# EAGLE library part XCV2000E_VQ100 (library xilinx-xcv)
xcv2000e_vq100 edit this description Auto generated by make-symbol-device-package-bsdl.ulp Rev. 26 Source: xcv2000e_vq100.bsd
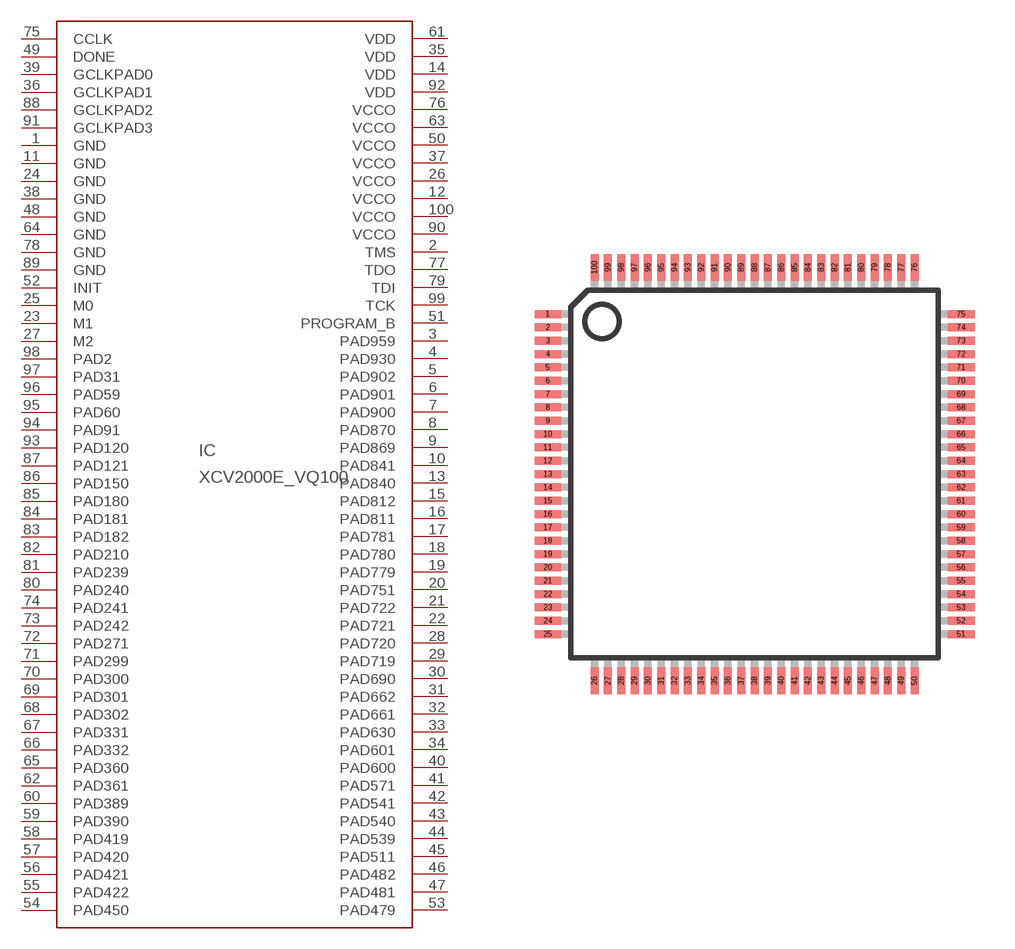
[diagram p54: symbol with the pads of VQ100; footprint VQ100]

Designator prefix IC

## XCV2000E_VQ100 (OC_FARNELL: unknown; OC_NEWARK: unknown)  [VQ100]
1  GND  pwr
2  TMS  in
3  PAD959
4  PAD930
5  PAD902
6  PAD901
7  PAD900
8  PAD870
9  PAD869
10  PAD841
11  GND  pwr
12  VCCO  pwr
13  PAD840
14  VDD  pwr
15  PAD812
16  PAD811
17  PAD781
18  PAD780
19  PAD779
20  PAD751
21  PAD722
22  PAD721
23  M1  in
24  GND  pwr
25  M0  in
26  VCCO  pwr
27  M2  in
28  PAD720
29  PAD719
30  PAD690
31  PAD662
32  PAD661
33  PAD630
34  PAD601
35  VDD  pwr
36  GCLKPAD1  in
37  VCCO  pwr
38  GND  pwr
39  GCLKPAD0  in
40  PAD600
41  PAD571
42  PAD541
43  PAD540
44  PAD539
45  PAD511
46  PAD482
47  PAD481
48  GND  pwr
49  DONE
50  VCCO  pwr
51  PROGRAM_B  in
52  INIT
53  PAD479
54  PAD450
55  PAD422
56  PAD421
57  PAD420
58  PAD419
59  PAD390
60  PAD389
61  VDD  pwr
62  PAD361
63  VCCO  pwr
64  GND  pwr
65  PAD360
66  PAD332
67  PAD331
68  PAD302
69  PAD301
70  PAD300
71  PAD299
72  PAD271
73  PAD242
74  PAD241
75  CCLK
76  VCCO  pwr
77  TDO  out
78  GND  pwr
79  TDI  in
80  PAD240
81  PAD239
82  PAD210
83  PAD182
84  PAD181
85  PAD180
86  PAD150
87  PAD121
88  GCLKPAD2  in
89  GND  pwr
90  VCCO  pwr
91  GCLKPAD3  in
92  VDD  pwr
93  PAD120
94  PAD91
95  PAD60
96  PAD59
97  PAD31
98  PAD2
99  TCK  in
100  VCCO  pwr

## Footprint VQ100 (pad centres in mm)
VQ100 Auto generated by make-symbol-device-package-bsdl.ulp Rev. 26
smd 1 x 0.3: 1 -7.75,6; 2 -7.75,5.5; 3 -7.75,5; 4 -7.75,4.5; 5 -7.75,4; 6 -7.75,3.5; 7 -7.75,3; 8 -7.75,2.5; 9 -7.75,2; 10 -7.75,1.5; 11 -7.75,1; 12 -7.75,0.5; 13 -7.75,0; 14 -7.75,-0.5; 15 -7.75,-1; 16 -7.75,-1.5; 17 -7.75,-2; 18 -7.75,-2.5; 19 -7.75,-3; 20 -7.75,-3.5; 21 -7.75,-4; 22 -7.75,-4.5; 23 -7.75,-5; 24 -7.75,-5.5; 25 -7.75,-6; 51 7.75,-6; 52 7.75,-5.5; 53 7.75,-5; 54 7.75,-4.5; 55 7.75,-4; 56 7.75,-3.5; 57 7.75,-3; 58 7.75,-2.5; 59 7.75,-2; 60 7.75,-1.5; 61 7.75,-1; 62 7.75,-0.5; 63 7.75,0; 64 7.75,0.5; 65 7.75,1; 66 7.75,1.5; 67 7.75,2; 68 7.75,2.5; 69 7.75,3; 70 7.75,3.5; 71 7.75,4; 72 7.75,4.5; 73 7.75,5; 74 7.75,5.5; 75 7.75,6
smd 0.3 x 1: 26 -6,-7.75; 27 -5.5,-7.75; 28 -5,-7.75; 29 -4.5,-7.75; 30 -4,-7.75; 31 -3.5,-7.75; 32 -3,-7.75; 33 -2.5,-7.75; 34 -2,-7.75; 35 -1.5,-7.75; 36 -1,-7.75; 37 -0.5,-7.75; 38 0,-7.75; 39 0.5,-7.75; 40 1,-7.75; 41 1.5,-7.75; 42 2,-7.75; 43 2.5,-7.75; 44 3,-7.75; 45 3.5,-7.75; 46 4,-7.75; 47 4.5,-7.75; 48 5,-7.75; 49 5.5,-7.75; 50 6,-7.75; 76 6,7.75; 77 5.5,7.75; 78 5,7.75; 79 4.5,7.75; 80 4,7.75; 81 3.5,7.75; 82 3,7.75; 83 2.5,7.75; 84 2,7.75; 85 1.5,7.75; 86 1,7.75; 87 0.5,7.75; 88 0,7.75; 89 -0.5,7.75; 90 -1,7.75; 91 -1.5,7.75; 92 -2,7.75; 93 -2.5,7.75; 94 -3,7.75; 95 -3.5,7.75; 96 -4,7.75; 97 -4.5,7.75; 98 -5,7.75; 99 -5.5,7.75; 100 -6,7.75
